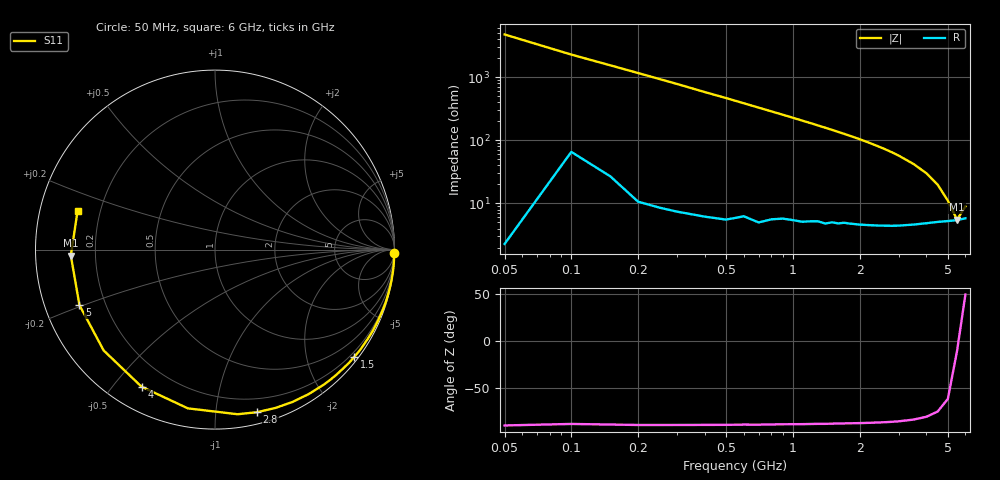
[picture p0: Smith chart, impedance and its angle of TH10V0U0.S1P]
! SIEMENS Discrete & RF Semiconductors
! BAS70
! Si Schottky Diode in SOT23
! VR = 10 V
! S-Parameters:  February  1997
# GHz  S  MA  R  50
!  f  S11
! GHz  MAG  ANG
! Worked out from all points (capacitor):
!   34 points, 50 MHz to 6 GHz, reference 50 ohm
!   read as one part to ground: C = 685 fF near 50 MHz
!   lowest |Z| = 5.54 ohm at 5.5 GHz (marker M1)
!   series resonance near 5.566 GHz, so ESL is about 1.2 nH
!   S11 on the Smith chart (normalised r, x): 50 MHz: 0, -95; 1.5 GHz: 0.10, -2.93; 2.8 GHz: 0.09, -1.29; 4 GHz: 0.10, -0.59; 5 GHz: 0.11, -0.20; 6 GHz: 0.12, +0.14
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0.05  1 -1.2
0.1  0.9988 -2.5
0.25  0.999 -6.1
0.4  0.9982 -9.8
0.5  0.9975 -12.2
0.6  0.9959 -14.7
0.7  0.9955 -17.2
0.8  0.9935 -19.7
1  0.9901 -24.7
1.1  0.9886 -27.3
1.2  0.9863 -29.8
1.4  0.9828 -35.0
1.5  0.9794 -37.6
1.6  0.9773 -40.3
1.7  0.9739 -42.9
1.8  0.9715 -45.7
2  0.9661 -51.2
2.2  0.9595 -57.0
2.4  0.9523 -63.0
2.6  0.9444 -69.1
2.8  0.9358 -75.5
3  0.9258 -82.2
3.5  0.8973 -99.7
4  0.8664 -118.2
4.5  0.837 -137.8
5  0.8162 -157.7
5.5  0.8039 -177.6
6  0.7955 164.3
